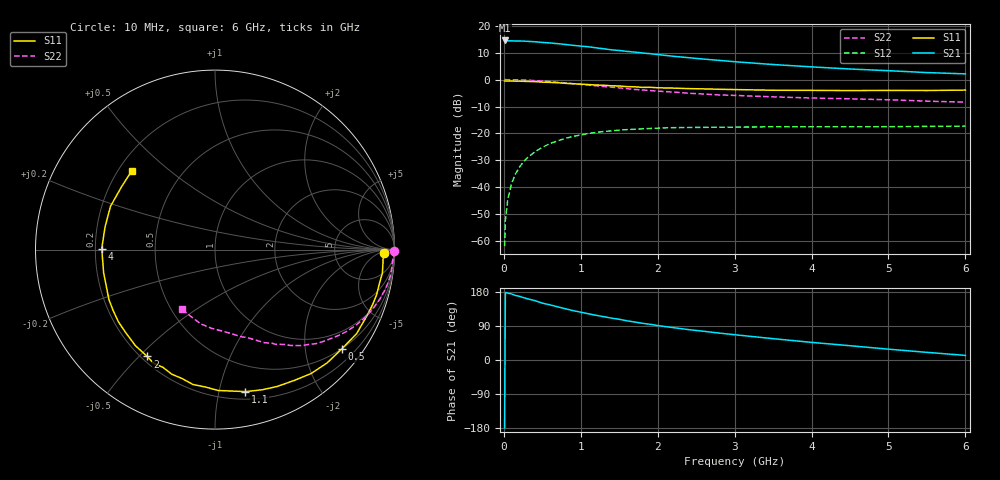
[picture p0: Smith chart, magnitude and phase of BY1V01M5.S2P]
! SIEMENS Small Signal Semiconductors
! BFY420
! Si NPN RF SIEGET Grounded Emitter Transistor in MICRO-X
! VCE = 1 V  IC = 1.5 mA
! Common Emitter S-Parameters:  October  1996
# GHz  S  MA  R  50
!  f  S11  S21  S12  S22
! GHz  MAG  ANG  MAG  ANG  MAG  ANG  MAG  ANG
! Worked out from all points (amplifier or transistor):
!   36 points, 10 MHz to 6 GHz, reference 50 ohm
!   highest |S21| = 14.6 dB at 10 MHz (marker M1)
!   |S21| within 3 dB of that: start of sweep to 1.273 GHz
!   unconditionally stable (mu >= 1): 4.236 GHz to end of sweep
!   at 250 MHz: K = 0.05, MSG = 22.5 dB, |S12| = -30.8 dB
!   at 1.4 GHz: K = 0.27, MSG = 15.1 dB, |S12| = -19.0 dB
!   at 6 GHz: K = 1.30, MAG = 6.4 dB, |S12| = -17.3 dB
!   S11 on the Smith chart (normalised r, x): 10 MHz: 30, -10; 500 MHz: 0.49, -2.81; 1.1 GHz: 0.26, -1.20; 2 GHz: 0.22, -0.53; 4 GHz: 0.23, +0.00; 6 GHz: 0.25, +0.38
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0.01  0.9413 -1.1  5.345 -179.5  0.0008 108.0  0.9966 -0.4
0.02  0.9378 -1.8  5.328 178.5  0.0024 88.3  0.9989 -0.8
0.05  0.9384 -4.0  5.257 176.5  0.0058 88.3  0.9953 -2.1
0.1  0.9418 -8.0  5.256 174.4  0.0116 84.9  0.9905 -4.3
0.15  0.9352 -11.6  5.22 170.3  0.0175 82.6  0.9899 -6.5
0.2  0.9348 -15.6  5.226 168.2  0.0233 80.9  0.9878 -8.4
0.25  0.9302 -19.2  5.204 164.9  0.029 77.7  0.9818 -10.7
0.4  0.9176 -30.7  5.062 156.8  0.0451 71.3  0.9583 -16.8
0.5  0.897 -38.2  4.919 150.2  0.0551 67.1  0.939 -20.7
0.7  0.8741 -52.1  4.66 140.3  0.073 58.9  0.8928 -28.0
0.8  0.8525 -58.7  4.497 135.2  0.0809 54.4  0.8678 -31.4
1.1  0.8091 -77.9  4.074 122.0  0.0997 44.3  0.7911 -40.3
1.4  0.7677 -93.9  3.575 110.5  0.1116 35.8  0.7237 -47.6
1.6  0.7409 -104.5  3.346 103.4  0.1177 31.1  0.6798 -51.8
2  0.7048 -122.4  2.921 90.9  0.1252 23.3  0.6101 -58.7
2.2  0.695 -129.7  2.719 85.5  0.1279 20.0  0.5876 -62.0
2.8  0.6614 -149.0  2.278 71.0  0.1306 12.8  0.5189 -70.4
3.5  0.6339 -168.2  1.908 56.3  0.1328 7.1  0.4779 -78.8
4  0.631 179.5  1.724 46.5  0.1327 4.2  0.4546 -85.3
4.5  0.6255 168.4  1.575 37.7  0.1328 1.5  0.4396 -92.2
5.5  0.6274 146.2  1.351 20.2  0.1349 -1.0  0.3978 -109.1
6  0.6385 136.6  1.278 12.1  0.1367 -1.5  0.38 -118.8
